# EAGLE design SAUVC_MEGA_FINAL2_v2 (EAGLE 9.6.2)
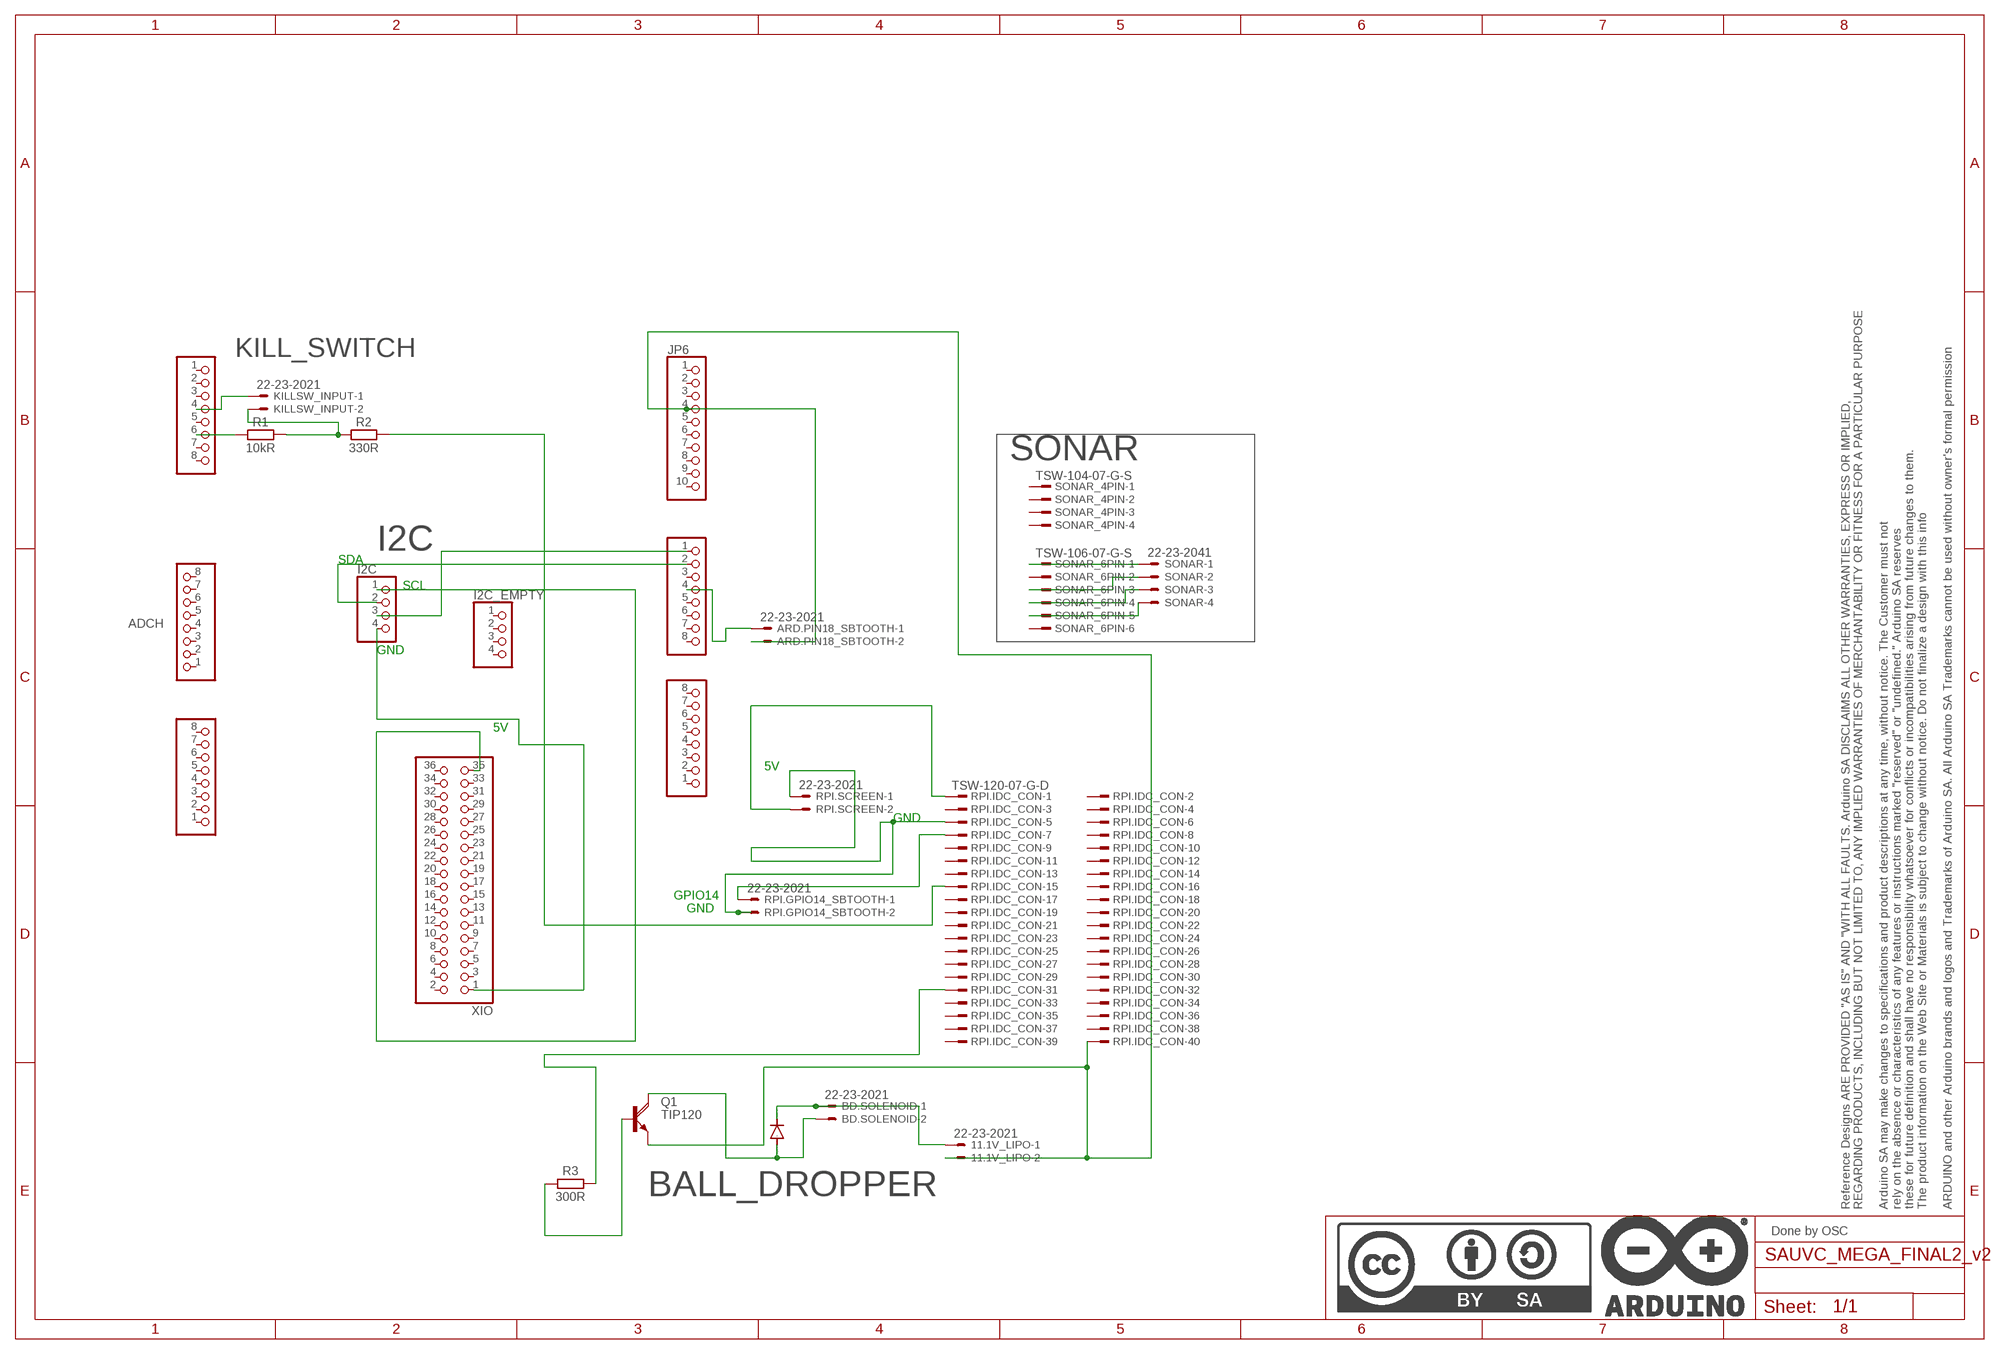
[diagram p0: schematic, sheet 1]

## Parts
1N5817  1N4004  [DO41-10]
11.1V_LIPO  22-23-2021  [22-23-2021]
ADCH  FH254-108DF08500V  0058_FH254-108DF08500V  [1X08]
ADCL  FH254-108DF08500V  0058_FH254-108DF08500V  [1X08]
ARD.PIN18_SBTOOTH  22-23-2021  [22-23-2021]
BD.SOLENOID  22-23-2021  [22-23-2021]
COMMUNICATION  FH254-108DF08500V  0058_FH254-108DF08500V  [1X08]
I2C  PINHD-1X4  [1X04]
I2C_EMPTY  PINHD-1X4  [1X04]
JP6  FH254-110DF08500V  1216_FH254-110DF08500T30  [1X10]
KILLSW_INPUT  22-23-2021  [22-23-2021]
POWER  FH254-108DF08500V  1217_FH254-108DF08500T21  [1X08]
PWML  FH254-108DF08500V  1218_FH254-108DF08500T20  [1X08]
Q1  TIP120  [TO220AH]
R1  10kR  R_AXIAL-7.2MM-PITCH  [RESAD724W46L381D178B]
R2  330R  R_AXIAL-7.2MM-PITCH  [RESAD724W46L381D178B]
R3  300R  R_AXIAL-7.2MM-PITCH  [RESAD724W46L381D178B]
RPI.GPIO14_SBTOOTH  22-23-2021  [22-23-2021]
RPI.IDC_CON  TSW-120-07-G-D  [TSW-120-XX-G-D]
RPI.SCREEN  22-23-2021  [22-23-2021]
SONAR  22-23-2041  [22-23-2041]
SONAR_4PIN  TSW-104-07-G-S  [TSW-104-XX-G-S]
SONAR_6PIN  TSW-106-07-G-S  [TSW-106-XX-G-S]
U$1  DNP  A3-FRAME  [FRAME]
XIO  18x2F-H8.5  0060_FH254-218DF08500V  [2X18]

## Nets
N$1: R2.2 RPI.IDC_CON.15
N$2: COMMUNICATION.1 I2C.3
N$3: COMMUNICATION.2 I2C.2
N$4: 1N5817.C 11.1V_LIPO.1 BD.SOLENOID.1
N$5: ARD.PIN18_SBTOOTH.1 COMMUNICATION.4
N$6: RPI.IDC_CON.1 RPI.SCREEN.2
N$7: 11.1V_LIPO.2 ARD.PIN18_SBTOOTH.2 JP6.4 Q1.E RPI.IDC_CON.40
N$8 [gnd]: Q1.B R3.1
N$9: KILLSW_INPUT.2 R1.2 R2.1
N$10: I2C.1 XIO.35
N$11: SONAR.1 SONAR_6PIN.1
N$12: I2C.4 XIO.1
N$13: SONAR.2 SONAR_6PIN.3
N$14: RPI.GPIO14_SBTOOTH.1 RPI.IDC_CON.7
N$16: RPI.GPIO14_SBTOOTH.2 RPI.IDC_CON.5 RPI.SCREEN.1
N$18: SONAR.3 SONAR_6PIN.4
N$19: SONAR.4 SONAR_6PIN.5
N$21: R3.2 RPI.IDC_CON.31
N$22: 1N5817.A BD.SOLENOID.2 Q1.C
N$24: KILLSW_INPUT.1 POWER.4
N$25: POWER.6 R1.1
Unconnected: ADCH.1 ADCH.2 ADCH.3 ADCH.4 ADCH.5 ADCH.6 ADCH.7 ADCH.8 ADCL.1 ADCL.2 ADCL.3 ADCL.4 ADCL.5 ADCL.6 ADCL.7 ADCL.8 COMMUNICATION.3 COMMUNICATION.5 COMMUNICATION.6 COMMUNICATION.7 COMMUNICATION.8 I2C_EMPTY.1 I2C_EMPTY.2 I2C_EMPTY.3 I2C_EMPTY.4 JP6.1 JP6.2 JP6.3 JP6.5 JP6.6 JP6.7 JP6.8 JP6.9 JP6.10 POWER.1 POWER.2 POWER.3 POWER.5 POWER.7 POWER.8 PWML.1 PWML.2 PWML.3 PWML.4 PWML.5 PWML.6 PWML.7 PWML.8 RPI.IDC_CON.2 RPI.IDC_CON.3 RPI.IDC_CON.4 RPI.IDC_CON.6 RPI.IDC_CON.8 RPI.IDC_CON.9 RPI.IDC_CON.10 RPI.IDC_CON.11 RPI.IDC_CON.12 RPI.IDC_CON.13 RPI.IDC_CON.14 RPI.IDC_CON.16 RPI.IDC_CON.17 RPI.IDC_CON.18 RPI.IDC_CON.19 RPI.IDC_CON.20 RPI.IDC_CON.21 RPI.IDC_CON.22 RPI.IDC_CON.23 RPI.IDC_CON.24 RPI.IDC_CON.25 RPI.IDC_CON.26 RPI.IDC_CON.27 RPI.IDC_CON.28 RPI.IDC_CON.29 RPI.IDC_CON.30 RPI.IDC_CON.32 RPI.IDC_CON.33 RPI.IDC_CON.34 RPI.IDC_CON.35 RPI.IDC_CON.36 RPI.IDC_CON.37 RPI.IDC_CON.38 RPI.IDC_CON.39 SONAR_4PIN.1 SONAR_4PIN.2 SONAR_4PIN.3 SONAR_4PIN.4 SONAR_6PIN.2 SONAR_6PIN.6 XIO.2 XIO.3 XIO.4 XIO.5 XIO.6 XIO.7 XIO.8 XIO.9 XIO.10 XIO.11 XIO.12 XIO.13 XIO.14 XIO.15 XIO.16 XIO.17 XIO.18 XIO.19 XIO.20 XIO.21 XIO.22 XIO.23 XIO.24 XIO.25 XIO.26 XIO.27 XIO.28 XIO.29 XIO.30 XIO.31 XIO.32 XIO.33 XIO.34 XIO.36

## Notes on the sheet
- KILL_SWITCH
- SONAR
- I2C
- SDA
- SCL
- GND
- 5V
- 5V
- GND
- GPIO14
- GND
- BALL_DROPPER
- Done by OSC

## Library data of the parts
1N5817 = diode:1N4004: DIODE
11.1V_LIPO ARD.PIN18_SBTOOTH BD.SOLENOID KILLSW_INPUT RPI.GPIO14_SBTOOTH RPI.SCREEN = con-molex:22-23-2021: .100" (2.54mm) Center Header - 2 Pin; MF: MOLEX; MPN: 22-23-2021; OC_FARNELL: 1462926; OC_NEWARK: 25C3832
ADCH ADCL COMMUNICATION = Connettori:0058_FH254-108DF08500V: Female Connector strip for Arduino bases - 8x1 F V h 8,5 p2,54mm; MONTHLY_USAGE: _____; PART_NUMBER: FH254-108DF08500V; PRICE: _____; SUPPLIER: _____; TYPE: Connettori
I2C I2C_EMPTY = pinhead:PINHD-1X4: PIN HEADER
JP6 = Connettori:1216_FH254-110DF08500T30: Female Connector strip for Arduino bases - 10x1 F V h 8,5 p2,54 serigrafato STRISCIA VUOTA; MONTHLY_USAGE: _____; PART_NUMBER: FH254-110DF08500T30; PRICE: _____; SUPPLIER: _____; TYPE: Connettori; VALUE: FH254-110DF08500T30
POWER = Connettori:1217_FH254-108DF08500T21: Female Connector strip for Arduino bases - 8x1 F V h 8,5 p2,54 serigrafato POWER; MONTHLY_USAGE: _____; PART_NUMBER: FH254-108DF08500T21; PRICE: _____; SUPPLIER: _____; TYPE: Connettori; VALUE: FH254-108DF08500T21
PWML = Connettori:1218_FH254-108DF08500T20: Female Connector strip for Arduino bases - 8x1 F V h 8,5 p2,54 serigrafato DIGITAL; MONTHLY_USAGE: _____; PART_NUMBER: FH254-108DF08500T20; PRICE: _____; SUPPLIER: _____; TYPE: Connettori; VALUE: FH254-108DF08500T20
Q1 = transistor-power:TIP120: NPN DARLINGTON TRANSISTOR
R1-R3 = Resistor:R: Resistor Fixed - Generic; CATEGORY: Resistor; SUB-CATEGORY: Fixed
RPI.IDC_CON = con-samtec:TSW-120-*-G: THROUGH-HOLE .025" SQ POST HEADER Source: Samtec TSW.pdf; MF: Samtec Inc.; MPN: TSW-120-07-G-D
SONAR = con-molex:22-23-2041: .100" (2.54mm) Center Header - 4 Pin; MF: MOLEX; MPN: 22-23-2041; OC_FARNELL: 1462920; OC_NEWARK: 38C0355
SONAR_4PIN = con-samtec:TSW-104-*-G-S: THROUGH-HOLE .025" SQ POST HEADER Source: Samtec TSW.pdf; MF: Samtec Inc.; MPN: TSW-104-07-G-S
SONAR_6PIN = con-samtec:TSW-106-*-G-S: THROUGH-HOLE .025" SQ POST HEADER Source: Samtec TSW.pdf; MF: Samtec Inc.; MPN: TSW-106-07-G-S
U$1 = Arduino-utility:A3-FRAME; CODE-ARDUINO: DNP; DATASHEET: DNP; DISTRIBUTOR-LINK: DNP; DISTRIBUTOR-PN: DNP; MANUFACTURER: DNP; MANUFACTURER-PN: DNP; NOTE: DNP
XIO = Connettori:0060_FH254-218DF08500V: 18x2 F V h 8,5 p2,54; MONTHLY_USAGE: _____; PART_NUMBER: FH254-218DF08500V; PRICE: _____; SUPPLIER: _____; TYPE: Connettori

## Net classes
0 default: width 0.203 mm, drill 0.406 mm, clearance 0.203 mm
1 power: width 0.61 mm, drill 0.406 mm, clearance 0.203 mm
2 gnd: width 0.305 mm, drill 0.406 mm, clearance 0.203 mm
3 power usb: width 0.508 mm, drill 0.406 mm, clearance 0.203 mm

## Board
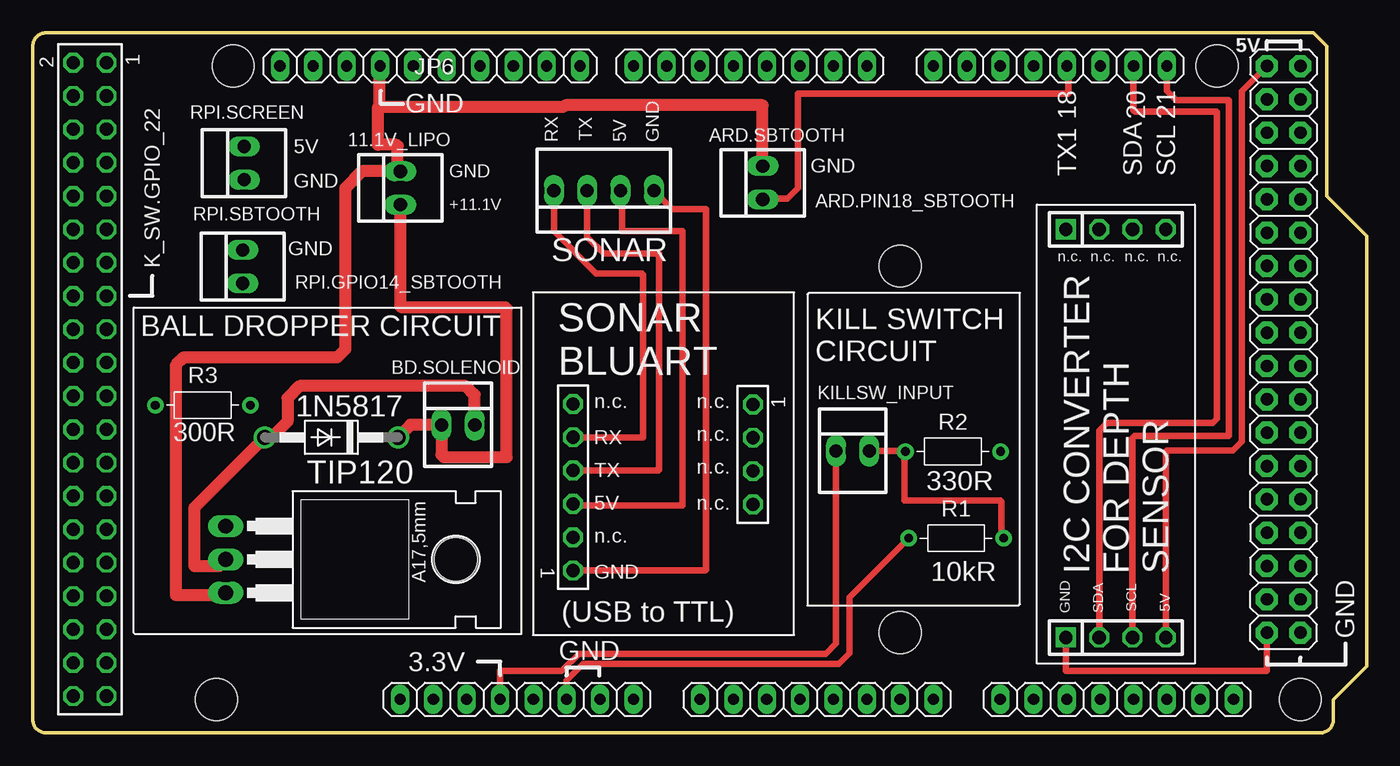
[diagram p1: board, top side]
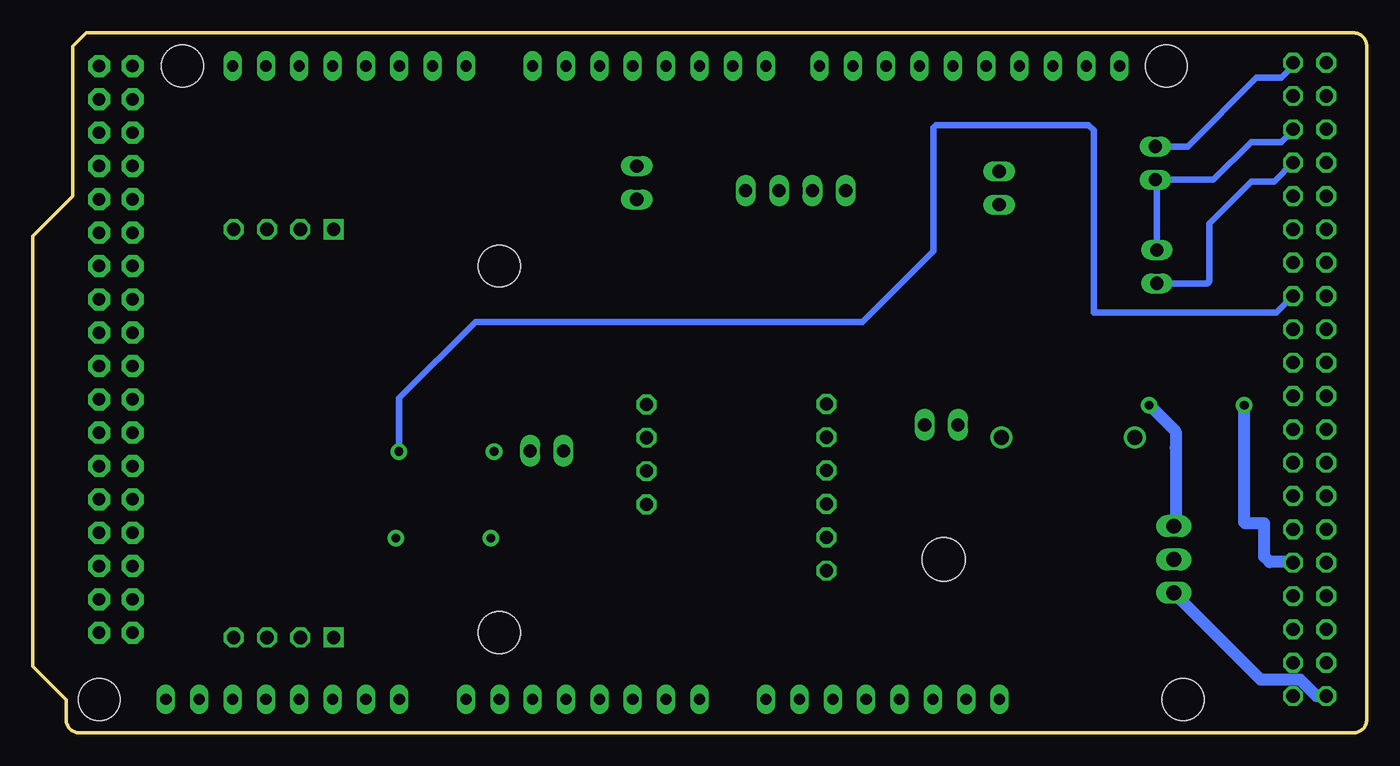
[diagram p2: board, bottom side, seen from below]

Size 101.6 x 53.34 mm. Coordinates in mm from the lower left corner, seen from the top.
Outline: 97.54,53.34 98.56,52.32 98.56,40.89 101.6,37.85 101.6,5.08 99.06,2.54 99.06,1 arc-90 98.06,0 1,0 arc-90 0,1 0,52.34 arc-90 1,53.34 97.54,53.34
Copper layers (1*16): Top 0.035mm / dielectric 1.5mm / Bottom 0.035mm
Design rules "ArduinoMega *": minimum track width 20mil, minimum drill 0.6mm, track to track 10mil, track to pad 10mil, pad to pad 10mil, via to via 10mil, smd to smd 7mil, copper to edge 27mil, drill to drill 12mil, minimum pad ring 10mil, minimum via ring 10mil, stop-mask expansion 2mil, vias tented up to drill 24mil, thermal gap 15mil
Holes 3.2 mm at 96.55,2.55 15.27,50.81 90.2,50.81 14,2.55 66.07,35.57 66.07,7.63

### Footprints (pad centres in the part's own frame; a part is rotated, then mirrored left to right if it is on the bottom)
DO41-10 = drill 1.118: A 5.08,0; C -5.08,0
22-23-2021 = drill 1 long: 1 -1.27,0; 2 1.27,0
1X08 = drill 0.85 pad 1.422 long: 1 -8.89,0; 2 -6.35,0; 3 -3.81,0; 4 -1.27,0; 5 1.27,0; 6 3.81,0; 7 6.35,0; 8 8.89,0
1X04 = drill 1.016 square: 1 -3.81,0 | drill 1.016 octagon: 2 -1.27,0; 3 1.27,0; 4 3.81,0
1X10 = drill 0.85 pad 1.422 long: 1 -11.43,0; 2 -8.89,0; 3 -6.35,0; 4 -3.81,0; 5 -1.27,0; 6 1.27,0; 7 3.81,0; 8 6.35,0; 9 8.89,0; 10 11.43,0
TO220AH = drill 1.118 long: B -2.54,-6.35; C 0,-6.35; E 2.54,-6.35 | hole 3.302: 0,11.176
RESAD724W46L381D178B = drill 0.66 pad 1.26: 1 -3.62,0; 2 3.62,0
TSW-120-XX-G-D = drill 1 pad 1.5 octagon: 1 24.13,-1.27; 2 24.13,1.27; 3 21.59,-1.27; 4 21.59,1.27; 5 19.05,-1.27; 6 19.05,1.27; 7 16.51,-1.27; 8 16.51,1.27; 9 13.97,-1.27; 10 13.97,1.27; 11 11.43,-1.27; 12 11.43,1.27; 13 8.89,-1.27; 14 8.89,1.27; 15 6.35,-1.27; 16 6.35,1.27; 17 3.81,-1.27; 18 3.81,1.27; 19 1.27,-1.27; 20 1.27,1.27; 21 -1.27,-1.27; 22 -1.27,1.27; 23 -3.81,-1.27; 24 -3.81,1.27; 25 -6.35,-1.27; 26 -6.35,1.27; 27 -8.89,-1.27; 28 -8.89,1.27; 29 -11.43,-1.27; 30 -11.43,1.27; 31 -13.97,-1.27; 32 -13.97,1.27; 33 -16.51,-1.27; 34 -16.51,1.27; 35 -19.05,-1.27; 36 -19.05,1.27; 37 -21.59,-1.27; 38 -21.59,1.27; 39 -24.13,-1.27; 40 -24.13,1.27
22-23-2041 = drill 1 long: 1 -3.81,0; 2 -1.27,0; 3 1.27,0; 4 3.81,0
TSW-104-XX-G-S = drill 1 pad 1.5 octagon: 1 3.81,0; 2 1.27,0; 3 -1.27,0; 4 -3.81,0
TSW-106-XX-G-S = drill 1 pad 1.5 octagon: 1 6.35,0; 2 3.81,0; 3 1.27,0; 4 -1.27,0; 5 -3.81,0; 6 -6.35,0
2X18 = drill 0.95 pad 1.676 octagon: 1 -21.59,-1.27; 2 -21.59,1.27; 3 -19.05,-1.27; 4 -19.05,1.27; 5 -16.51,-1.27; 6 -16.51,1.27; 7 -13.97,-1.27; 8 -13.97,1.27; 9 -11.43,-1.27; 10 -11.43,1.27; 11 -8.89,-1.27; 12 -8.89,1.27; 13 -6.35,-1.27; 14 -6.35,1.27; 15 -3.81,-1.27; 16 -3.81,1.27; 17 -1.27,-1.27; 18 -1.27,1.27; 19 1.27,-1.27; 20 1.27,1.27; 21 3.81,-1.27; 22 3.81,1.27; 23 6.35,-1.27; 24 6.35,1.27; 25 8.89,-1.27; 26 8.89,1.27; 27 11.43,-1.27; 28 11.43,1.27; 29 13.97,-1.27; 30 13.97,1.27; 31 16.51,-1.27; 32 16.51,1.27; 33 19.05,-1.27; 34 19.05,1.27; 35 21.59,-1.27; 36 21.59,1.27

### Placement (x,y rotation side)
1N5817  22.74,22.51 180 top
11.1V_LIPO  27.99,41.51 90 top
ADCH  82.58,2.55 0 top
ADCL  59.72,2.55 0 top
ARD.PIN18_SBTOOTH  55.59,41.91 90 top
BD.SOLENOID  32.39,23.46 0 top
COMMUNICATION  77.5,50.81 180 top
I2C  82.49,7.26 0 top
I2C_EMPTY  82.49,38.36 0 top
JP6  30.25,50.81 0 top
KILLSW_INPUT  62.45,21.49 0 top
POWER  36.86,2.55 0 top
PWML  54.64,50.81 180 top
Q1  21.04,13.21 270 top
R1  70.32,14.83 0 top
R2  70.09,21.44 0 top
R3  12.94,24.96 180 top
RPI.GPIO14_SBTOOTH  15.99,35.52 90 top
RPI.IDC_CON  4.34,26.94 90 top
RPI.SCREEN  16.09,43.41 90 top
SONAR  43.49,41.31 180 top
SONAR_4PIN  54.84,21.21 90 top
SONAR_6PIN  41.14,18.71 270 top
U$1  0.03,0.01 0 top
XIO  95.28,29.22 270 top

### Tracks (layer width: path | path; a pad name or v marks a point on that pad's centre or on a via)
N$1
  Bottom 0.508: R2.2 73.71,25.5 67.89,31.31 38.39,31.31 32.99,36.71 32.99,46.11 32.79,46.31 21.19,46.31 20.79,45.91 20.79,32.01 6.89,32.01 RPI.IDC_CON.15
N$2
  Top 0.508: COMMUNICATION.1 86.39,48.92 87.09,48.21 91.09,48.21 91.09,22.61 83.89,22.61 83.76,22.48 I2C.3
N$3
  Top 0.508: COMMUNICATION.2 83.85,47.46 83.99,47.31 90.19,47.31 90.19,23.91 89.89,23.61 81.79,23.61 81.22,23.04 I2C.2
N$4
  Top 0.9: 1N5817.C 28.77,23.46 BD.SOLENOID.1 31.12,21.18 31.29,21.01 36.09,21.01 36.09,32.31 35.99,32.41 28.09,32.41 27.99,32.51 11.1V_LIPO.1
N$5
  Top 0.508: ARD.PIN18_SBTOOTH.1 55.66,40.71 57.49,40.71 58.29,41.51 58.29,48.71 78.89,48.71 78.89,50.68 COMMUNICATION.4
N$6
  Bottom 0.508: RPI.SCREEN.2 13.62,44.68 8.39,49.91 6.49,49.91 5.61,50.79 RPI.IDC_CON.1
N$7
  Top 0.508: JP6.4 26.39,50.76 | 14.53,10.51 Q1.E
  Top 0.9: 26.39,50.76 26.39,47.71 | 26.39,47.71 40.46,47.71 40.56,47.81 55.59,47.81 ARD.PIN18_SBTOOTH.2 | 26.39,47.71 26.29,47.61 26.29,44.81 27.69,44.81 27.79,44.71 27.79,42.98 11.1V_LIPO.2 25.06,42.78 23.79,41.51 23.79,29.21 23.19,28.61 11.49,28.61 10.89,28.01 10.89,10.51 14.53,10.51
  Bottom 0.508: 3.83,2.81 RPI.IDC_CON.40 | 14.63,10.61 Q1.E
  Bottom 0.9: Q1.E 8.09,4.07 5.09,4.07 3.83,2.81
N$8
  Bottom 0.508: 14.55,15.61 Q1.B
  Bottom 0.9: R3.1 14.55,22.95 14.55,21.71 | 14.55,21.71 14.55,15.61 | 14.55,21.71
N$9
  Top 0.508: KILLSW_INPUT.2 66.42,21.49 R2.1 66.39,21.36 66.39,17.71 73.69,17.71 73.79,17.61 73.79,14.97 R1.2
N$10
  Top 0.508: I2C.1 78.68,4.71 93.99,4.71 94.01,4.73 XIO.35
N$11
  Top 0.508: SONAR.1 48.7,39.91 51.29,39.91 51.29,12.41 51.24,12.36 SONAR_6PIN.1
N$12
  Top 0.508: XIO.1 92.09,48.9 92.09,22.21 91.39,21.51 86.39,21.51 86.3,21.42 I2C.4
N$13
  Top 0.508: SONAR.2 44.89,41.18 44.89,38.21 49.49,38.21 49.49,17.31 41.27,17.31 SONAR_6PIN.3
N$14
  Bottom 0.508: RPI.IDC_CON.7 7.05,42.01 8.79,42.01 11.99,38.81 11.99,34.41 12.16,34.25 RPI.GPIO14_SBTOOTH.1
N$16
  Bottom 0.508: RPI.GPIO14_SBTOOTH.2 15.99,42.04 RPI.SCREEN.1 11.66,42.14 8.79,45.01 6.49,45.01 5.61,45.89 RPI.IDC_CON.5
N$18
  Top 0.508: SONAR.3 42.22,37.78 43.49,36.51 47.69,36.51 47.69,20.01 47.66,19.98 SONAR_6PIN.4
N$19
  Top 0.508: SONAR.4 39.68,38.22 42.89,35.01 46.39,35.01 46.49,34.91 46.49,22.51 SONAR_6PIN.5
N$21
  Bottom 0.9: R3.2 9.32,16.04 9.25,15.97 7.81,15.97 7.81,13.43 7.39,13.01 5.66,13.01 RPI.IDC_CON.31
N$22
  Top 0.9: BD.SOLENOID.2 33.66,25.74 32.99,26.41 20.29,26.41 19.39,25.51 19.39,23.71 18.19,22.51 1N5817.A 12.29,17.14 12.29,12.71 14.19,12.71 Q1.C
N$24
  Top 0.508: KILLSW_INPUT.1 61.18,6.8 60.42,6.04 41.61,6.04 40.29,4.71 35.59,4.71 POWER.4
N$25
  Top 0.508: POWER.6 40.67,4.01 41.93,5.28 61.41,5.28 62.19,6.06 62.19,10.32 R1.1

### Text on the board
tPlace: 18 | 20 | 21
tNames: 5V | GND | RX | TX | 5V | GND | ARD.SBTOOTH | 5V | GND | GND | TX1 | SDA | SCL | GND | +11.1V | RPI.SBTOOTH | GND | n.c. | n.c. | n.c. | n.c. | SONAR | K_SW.GPIO_22 | BALL DROPPER CIRCUIT | KILL SWITCH / CIRCUIT | n.c. | n.c. | 1N5817 | SONAR / BLUART | 300R | RX | n.c. | n.c. | TX | 330R | 5V | n.c. | n.c. | GND | 10kR | I2C CONVERTER / FOR DEPTH / SENSOR | GND | SDA | SCL | 5V | (USB to TTL) | GND | GND | 3.3V
tValues: MEGA 2560 / SAUVC 20/21

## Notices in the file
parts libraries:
Arduino-utility: Copyright (c) 2016-2017 Arduino LLC. All right reserved.
